(* Logix 5000 AddOnInstructionDefinition export AMCI_SV160E2_Axis_Follower_Linear; software revision 20.03 *)

ADD_ON_INSTRUCTION AMCI_SV160E2_Axis_Follower_Linear   (* revision 1.0, vendor AMCI, ExecuteEnableInFalse *)
// Revision note:
// 8/2019 Version 0 Initial release of SV160E2 Add On Instructions.
// 3/72020 Version 1 3/17/20 Version 1 replaced the generic EDS file with a more complete V1.6 EDS file.  Also added a line of code to limit the minimum follower acceleration to -15999.
// Help:
// 2/2017: V0 is the initial release
// 7/2017: V1 added enable and error bits.
// 5/2019: V2 added unlatching the error bit when the rung goes false and the ability to select between normal (jog CCW) and continuous follower (jog CW)
VAR_OUTPUT
   EN : BOOL; {visible}
END_VAR
VAR_INPUT
   Status_Word_0 : INT; {required}
        .0   // set when moving CW
        .1   // set when moving CCW
        .3   // set when stopped
   Status_Word_1 : INT; {required}
        .15   // 0 when disabled 1 when enabled
   Follower_Position : REAL; {required}
   Follower_Velocity : REAL; {required}
   Follower_Acceleration : REAL; {required}
   Ramp_Acceleration : INT; {required}
   Deceleration : INT; {required}
   Maximum_Move_Torque : INT;
END_VAR
VAR_IN_OUT
   AMCI_SV160E2_output_data : _000A:SV160E2_9125ACD4:O:0; {required}
END_VAR
VAR_OUTPUT
   Axis_Follower_occurring : BOOL; {visible}
   ER : BOOL; {visible}
END_VAR
VAR
   command_data_block : INT[10];
        [0]   // Command Bits MSW
        [1]   // Command Bits LSW
        [2]   // Upper Target Position
        [3]   // Lower Target Position
        [4]   // Upper Programmed Speed
        [5]   // Lower Programmed Speed
   axis_follower_position : DINT;
   axis_follower_velocity : DINT;
END_VAR

ROUTINE EnableInFalse   (* ladder *)
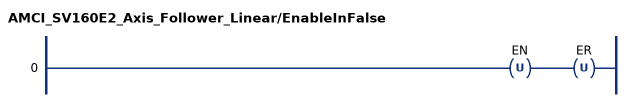
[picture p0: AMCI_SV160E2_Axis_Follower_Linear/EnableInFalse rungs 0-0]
   0: OTU(EN)OTU(ER);
END_ROUTINE

ROUTINE Logic   (* ladder *)
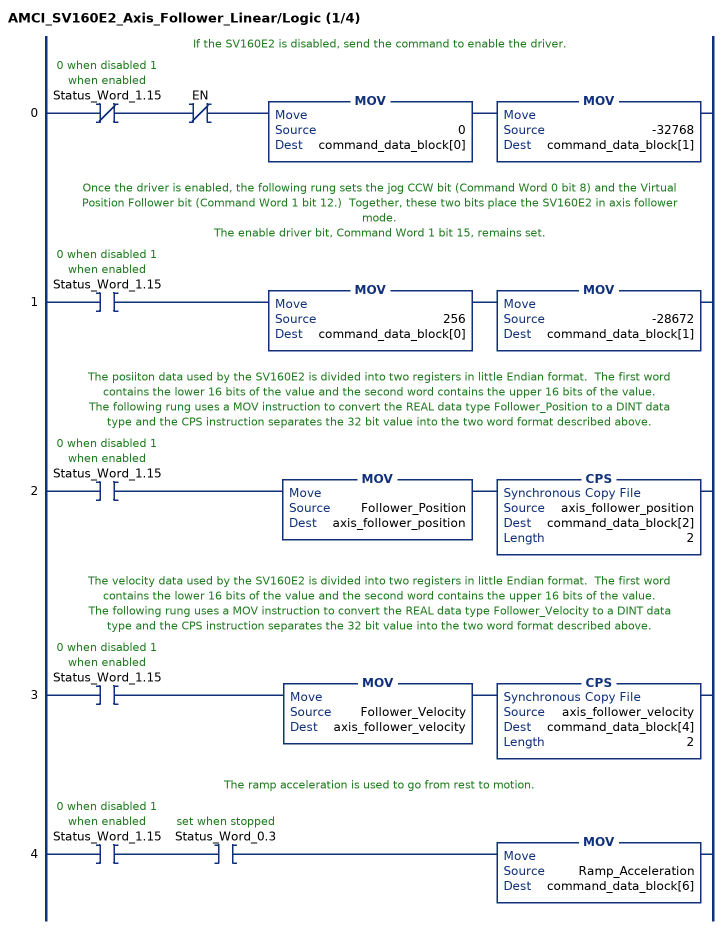
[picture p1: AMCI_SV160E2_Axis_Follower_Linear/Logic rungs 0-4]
   // If the SV160E2 is disabled, send the command to enable the driver.
   0: XIO(Status_Word_1.15)XIO(EN)MOV(0,command_data_block[0])MOV(-32768,command_data_block[1]);
   // Once the driver is enabled, the following rung sets the jog CCW bit (Command Word 0 bit 8) and the Virtual Position Follower bit (Command Word 1 bit 12.)  Together, these two bits place the SV160E2 in axis follower mode.
   // The enable driver bit, Command Word 1 bit 15, remains set.
   1: XIC(Status_Word_1.15)MOV(256,command_data_block[0])MOV(-28672,command_data_block[1]);
   // The posiiton data used by the SV160E2 is divided into two registers in little Endian format.  The first word contains the lower 16 bits of the value and the second word contains the upper 16 bits of the value.
   // The following rung uses a MOV instruction to convert the REAL data type Follower_Position to a DINT data type and the CPS instruction separates the 32 bit value into the two word format described above.
   2: XIC(Status_Word_1.15)MOV(Follower_Position,axis_follower_position)CPS(axis_follower_position,command_data_block[2],2);
   // The velocity data used by the SV160E2 is divided into two registers in little Endian format.  The first word contains the lower 16 bits of the value and the second word contains the upper 16 bits of the value.
   // The following rung uses a MOV instruction to convert the REAL data type Follower_Velocity to a DINT data type and the CPS instruction separates the 32 bit value into the two word format described above.
   3: XIC(Status_Word_1.15)MOV(Follower_Velocity,axis_follower_velocity)CPS(axis_follower_velocity,command_data_block[4],2);
   // The ramp acceleration is used to go from rest to motion.
   4: XIC(Status_Word_1.15)XIC(Status_Word_0.3)MOV(Ramp_Acceleration,command_data_block[6]);
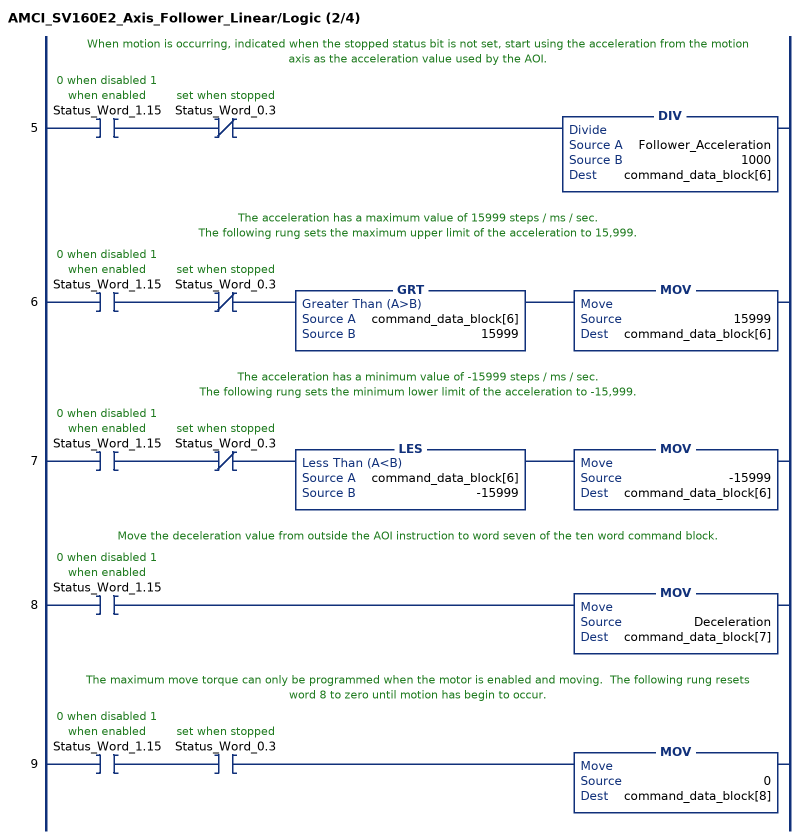
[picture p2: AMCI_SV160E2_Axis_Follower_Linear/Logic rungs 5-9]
   // When motion is occurring, indicated when the stopped status bit is not set, start using the acceleration from the motion axis as the acceleration value used by the AOI.
   5: XIC(Status_Word_1.15)XIO(Status_Word_0.3)DIV(Follower_Acceleration,1000,command_data_block[6]);
   // The acceleration has a maximum value of 15999 steps / ms / sec.
   // The following rung sets the maximum upper limit of the acceleration to 15,999.
   6: XIC(Status_Word_1.15)XIO(Status_Word_0.3)GRT(command_data_block[6],15999)MOV(15999,command_data_block[6]);
   // The acceleration has a minimum value of -15999 steps / ms / sec.
   // The following rung sets the minimum lower limit of the acceleration to -15,999.
   7: XIC(Status_Word_1.15)XIO(Status_Word_0.3)LES(command_data_block[6],-15999)MOV(-15999,command_data_block[6]);
   // Move the deceleration value from outside the AOI instruction to word seven of the ten word command block.
   8: XIC(Status_Word_1.15)MOV(Deceleration,command_data_block[7]);
   // The maximum move torque can only be programmed when the motor is enabled and moving.  The following rung resets word 8 to zero until motion has begin to occur.
   9: XIC(Status_Word_1.15)XIC(Status_Word_0.3)MOV(0,command_data_block[8]);
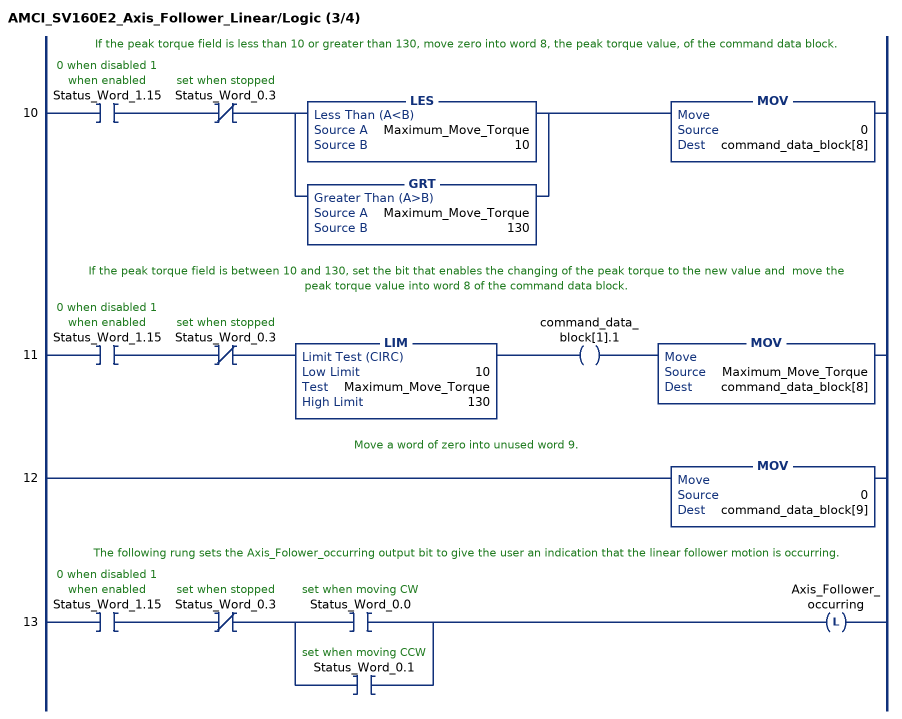
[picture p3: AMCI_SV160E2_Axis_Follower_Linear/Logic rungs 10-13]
   // If the peak torque field is less than 10 or greater than 130, move zero into word 8, the peak torque value, of the command data block.
   10: XIC(Status_Word_1.15)XIO(Status_Word_0.3)[LES(Maximum_Move_Torque,10) ,GRT(Maximum_Move_Torque,130) ]MOV(0,command_data_block[8]);
   // If the peak torque field is between 10 and 130, set the bit that enables the changing of the peak torque to the new value and  move the peak torque value into word 8 of the command data block.
   11: XIC(Status_Word_1.15)XIO(Status_Word_0.3)LIM(10,Maximum_Move_Torque,130)OTE(command_data_block[1].1)MOV(Maximum_Move_Torque,command_data_block[8]);
   // Move a word of zero into unused word 9.
   12: MOV(0,command_data_block[9]);
   // The following rung sets the Axis_Folower_occurring output bit to give the user an indication that the linear follower motion is occurring.
   13: XIC(Status_Word_1.15)XIO(Status_Word_0.3)[XIC(Status_Word_0.0) ,XIC(Status_Word_0.1) ]OTL(Axis_Follower_occurring);
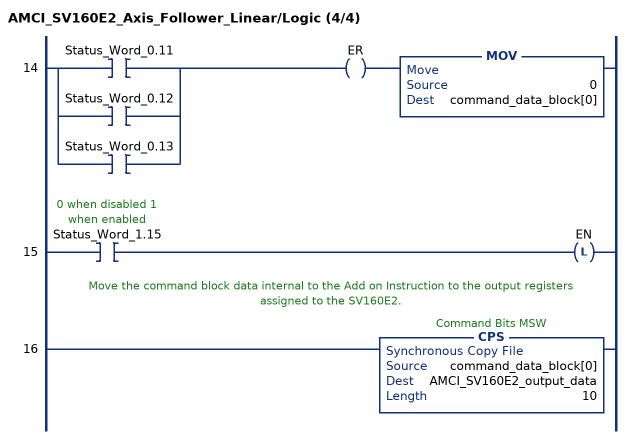
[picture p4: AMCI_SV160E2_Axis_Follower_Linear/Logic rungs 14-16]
   14: [XIC(Status_Word_0.11) ,XIC(Status_Word_0.12) ,XIC(Status_Word_0.13) ]OTE(ER)MOV(0,command_data_block[0]);
   15: XIC(Status_Word_1.15)OTL(EN);
   // Move the command block data internal to the Add on Instruction to the output registers assigned to the SV160E2.
   16: CPS(command_data_block[0],AMCI_SV160E2_output_data,10);
END_ROUTINE
END_ADD_ON_INSTRUCTION
